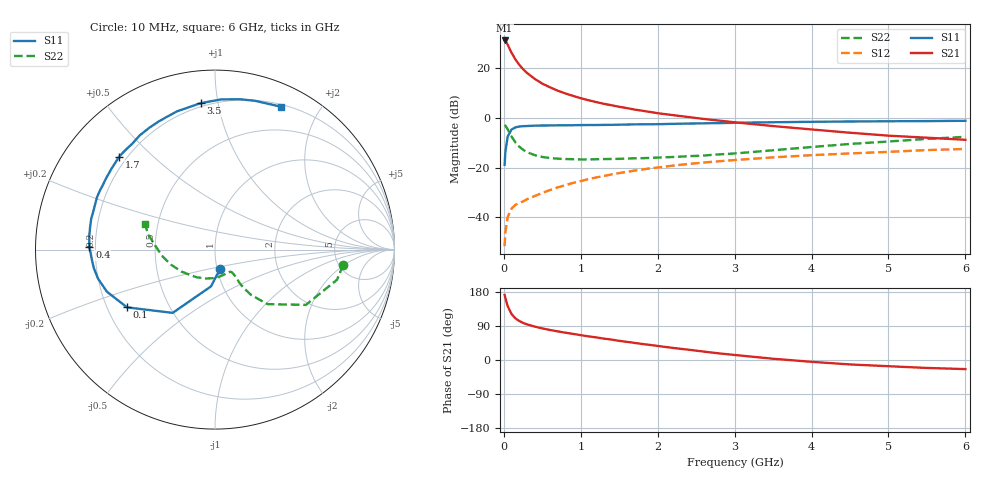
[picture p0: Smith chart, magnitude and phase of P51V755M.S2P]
! SIEMENS Small Signal Semiconductors
! BFP183
! Si NPN RF Bipolar Junction Transistor in SOT143
! VCE = 1.75 V  IC = 55 mA
! Common Emitter S-Parameters:  March  1996
# GHz  S  MA  R  50
!  f  S11  S21  S12  S22
! GHz  MAG  ANG  MAG  ANG  MAG  ANG  MAG  ANG
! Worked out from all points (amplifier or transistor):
!   36 points, 10 MHz to 6 GHz, reference 50 ohm
!   highest |S21| = 31.3 dB at 10 MHz (marker M1)
!   |S21| within 3 dB of that: start of sweep to 69.82 MHz
!   unconditionally stable (mu >= 1): start of sweep to 33.33 MHz; 182 MHz to end of sweep
!   at 250 MHz: K = 1.21, MAG = 23.9 dB, |S12| = -33.7 dB
!   at 1.4 GHz: K = 1.74, MAG = 8.9 dB, |S12| = -22.8 dB
!   at 6 GHz: K = 1.35, MAG = -1.7 dB, |S12| = -12.5 dB
!   S11 on the Smith chart (normalised r, x): 10 MHz: 1.03, -0.23; 100 MHz: 0.28, -0.28; 400 MHz: 0.18, +0.01; 1.7 GHz: 0.17, +0.39; 3.5 GHz: 0.18, +0.89; 6 GHz: 0.22, +1.54
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0.01  0.1135 -76.2  36.56 171.6  0.0026 65.5  0.7195 -6.8
0.02  0.2062 -96.2  35.64 163.4  0.005 63.5  0.7002 -13.9
0.05  0.4243 -123.8  29.99 142.1  0.0101 61.0  0.5928 -31.3
0.1  0.5862 -146.7  20.69 121.4  0.0149 46.5  0.4216 -46.1
0.15  0.6462 -158.7  15.2 110.0  0.0176 45.1  0.3226 -51.5
0.2  0.6712 -166.0  11.84 103.0  0.0194 46.5  0.2642 -53.3
0.25  0.683 -171.3  9.648 97.9  0.0207 48.5  0.2289 -53.6
0.3  0.6881 -175.2  8.133 94.2  0.0229 50.0  0.205 -53.1
0.4  0.6997 178.8  6.16 88.2  0.0266 54.0  0.1784 -52.8
0.5  0.7047 174.0  4.927 83.4  0.0309 55.9  0.1635 -53.1
0.6  0.707 169.8  4.156 79.2  0.0352 58.2  0.1557 -53.7
0.7  0.7108 166.1  3.547 75.5  0.0398 59.7  0.151 -55.0
0.9  0.7135 159.6  2.786 68.9  0.049 61.1  0.1473 -59.2
1.1  0.7208 152.9  2.28 62.4  0.0587 60.6  0.146 -64.2
1.3  0.7249 147.2  1.931 56.5  0.0677 59.9  0.1483 -69.9
1.7  0.7436 136.1  1.477 45.1  0.0869 57.3  0.1538 -82.9
2.2  0.7621 123.4  1.14 31.8  0.1094 52.4  0.1632 -100.9
2.8  0.7882 109.3  0.885 17.4  0.1341 46.0  0.1845 -123.1
3.5  0.8198 95.6  0.687 3.3  0.1604 38.6  0.2232 -146.8
4.5  0.849 80.7  0.504 -11.7  0.1926 27.7  0.2993 -173.8
5.5  0.8647 69.9  0.4 -21.0  0.2252 18.3  0.3784 167.8
6  0.8774 65.1  0.363 -24.0  0.2374 12.9  0.417 159.9
